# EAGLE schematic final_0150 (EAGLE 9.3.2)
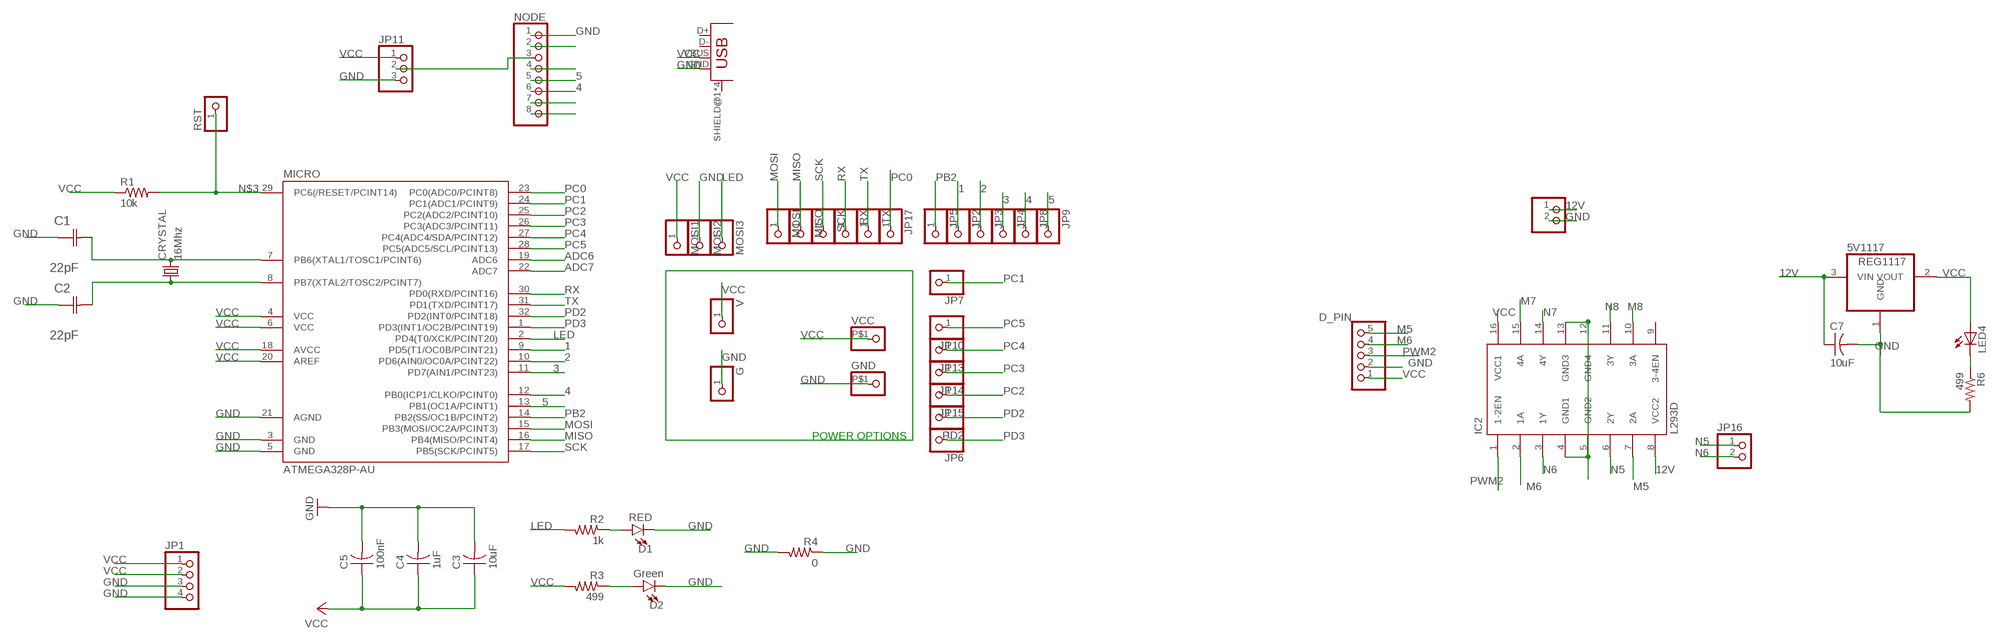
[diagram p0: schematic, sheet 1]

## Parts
5V1117  REG1117  [SOT223]
C1  22pF  0612ZC225MAT2A  [CAPC3216X178N]
C2  22pF  0612ZC225MAT2A  [CAPC3216X178N]
C3  10uF  CAP-US1206FAB  [C1206FAB]
C4  1uF  CAP-US1206FAB  [C1206FAB]
C5  100nF  CAP-US1206FAB  [C1206FAB]
C7  10uF  CAP-US1206FAB  [C1206FAB]
CRYSTAL  16Mhz  CSM-7X-DU  [CSM-7X-DU]
D1  RED  LED-RED1206  [LED-1206]
D2  Green  LED-RED1206  [LED-1206]
D_PIN  PINHD-1X5  [1X05]
G  PINHD-1X1  [1X01]
GND  PINHD-1X1-BIGPOGO  [1X1-BIGPOGO]
IC2  L293D  [DIL16]
JP1  PINHD-1X4  [1X04]
JP2  PINHD-1X1  [1X01]
JP3  PINHD-1X1  [1X01]
JP4  PINHD-1X1  [1X01]
JP5  PINHD-1X1  [1X01]
JP6  PINHD-1X1  [1X01]
JP7  PINHD-1X1  [1X01]
JP8  PINHD-1X1  [1X01]
JP9  PINHD-1X1  [1X01]
JP10  PINHD-1X1  [1X01]
JP11  PINHD-1X3  [1X03]
JP12  PINHD-1X2  [1X02]
JP13  PINHD-1X1  [1X01]
JP14  PINHD-1X1  [1X01]
JP15  PINHD-1X1  [1X01]
JP16  PINHD-1X2  [1X02]
JP17  PINHD-1X1  [1X01]
LED4  LEDSMT1206  [1206]
MICRO  ATMEGA328P-AU  ATMEGA48/88/168-AU  [TQFP32-08]
MISO  PINHD-1X1  [1X01]
MOSI  PINHD-1X1  [1X01]
MOSI1  PINHD-1X1  [1X01]
MOSI2  PINHD-1X1  [1X01]
MOSI3  PINHD-1X1  [1X01]
NODE  PINHD-1X8  [1X08]
PD2  PINHD-1X1  [1X01]
R1  10k  RES-US1206FAB  [R1206FAB]
R2  1k  RES-US1206FAB  [R1206FAB]
R3  499  RES-US1206FAB  [R1206FAB]
R4  0  RES-US1206FAB  [R1206FAB]
R6  499  RESISTOR1206  [1206]
RST  PINHD-1X1  [1X01]
RX  PINHD-1X1  [1X01]
SCK  PINHD-1X1  [1X01]
TX  PINHD-1X1  [1X01]
U$1  USB_MINIB  [USB_MINIB]
V  PINHD-1X1  [1X01]
VCC  PINHD-1X1-BIGPOGO  [1X1-BIGPOGO]

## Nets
1: JP2.1 MICRO.9(PD5(T1/OC0B/PCINT21))
2: JP3.1 MICRO.10(PD6(AIN0/OC0A/PCINT22))
3: JP4.1 MICRO.11(PD7(AIN1/PCINT23))
4: JP8.1 MICRO.12(PB0(ICP1/CLKO/PCINT0)) NODE.6
5: JP9.1 MICRO.13(PB1(OC1A/PCINT1)) NODE.5
12V: 5V1117.3(VIN) C7.1 IC2.8(VCC2) JP12.1
ADC6: MICRO.19(ADC6)
ADC7: MICRO.22(ADC7)
GND: 5V1117.1(GND) C1.1(C1) C2.1(C1) C3.2 C4.2 C5.2 C7.2 D1.C D2.C D_PIN.2 G.1 GND.P$1 IC2.4(GND1) IC2.5(GND2) IC2.12(GND4) IC2.13(GND3) JP1.3 JP1.4 JP11.3 JP12.2 MICRO.3(GND) MICRO.5(GND) MICRO.21(AGND) MOSI2.1 NODE.1 R4.1 R4.2 R6.2 U$1.GND
LED: MICRO.2(PD4(T0/XCK/PCINT20)) MOSI3.1 R2.2
M5: D_PIN.5 IC2.7(2A)
M6: D_PIN.4 IC2.2(1A)
M7: IC2.15(4A)
M8: IC2.10(3A)
MISO: MICRO.16(PB4(MISO/PCINT4)) MISO.1
MOSI: MICRO.15(PB3(MOSI/OC2A/PCINT3)) MOSI.1
N5: IC2.6(2Y) JP16.1
N6: IC2.3(1Y) JP16.2
N7: IC2.14(4Y)
N8: IC2.11(3Y)
N$1: D2.A R3.1
N$2: C1.2(C2) CRYSTAL.2 MICRO.7(PB6(XTAL1/TOSC1/PCINT6))
N$3: MICRO.29(PC6(/RESET/PCINT14)) R1.2 RST.1
N$4: LED4.C R6.1
N$5: NODE.2
N$7: NODE.4
N$8: JP11.2 NODE.3
N$9: C2.2(C2) CRYSTAL.1 MICRO.8(PB7(XTAL2/TOSC2/PCINT7))
N$11: NODE.7
N$12: NODE.8
N$25: D1.A R2.1
PB2: JP5.1 MICRO.14(PB2(SS/OC1B/PCINT2))
PC0: JP17.1 MICRO.23(PC0(ADC0/PCINT8))
PC1: JP7.1 MICRO.24(PC1(ADC1/PCINT9))
PC2: JP15.1 MICRO.25(PC2(ADC2/PCINT10))
PC3: JP14.1 MICRO.26(PC3(ADC3/PCINT11))
PC4: JP13.1 MICRO.27(PC4(ADC4/SDA/PCINT12))
PC5: JP10.1 MICRO.28(PC5(ADC5/SCL/PCINT13))
PD2: MICRO.32(PD2(INT0/PCINT18)) PD2.1
PD3: JP6.1 MICRO.1(PD3(INT1/OC2B/PCINT19))
PWM2: D_PIN.3 IC2.1(1-2EN)
RX: MICRO.30(PD0(RXD/PCINT16)) RX.1
SCK: MICRO.17(PB5(SCK/PCINT5)) SCK.1
TX: MICRO.31(PD1(TXD/PCINT17)) TX.1
VCC: 5V1117.2(VOUT) C3.1 C4.1 C5.1 D_PIN.1 IC2.16(VCC1) JP1.1 JP1.2 JP11.1 LED4.A MICRO.4(VCC) MICRO.6(VCC) MICRO.18(AVCC) MICRO.20(AREF) MOSI1.1 R1.1 R3.2 U$1.VBUS V.1 VCC.P$1
Unconnected: IC2.9(3-4EN) U$1.D+ U$1.D- U$1.SHIELD@1(SHIELD) U$1.SHIELD@2(SHIELD) U$1.SHIELD@3(SHIELD) U$1.SHIELD@4(SHIELD)

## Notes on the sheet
- POWER OPTIONS

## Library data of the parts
5V1117 = burr-brown:REG1117: 800mA and 1A Low Dropout (LDO) Positive Regulator 1.8V, 2.5V, 2.85V, 3.3V, 5V, and Adj; MPN: REG1117; OC_FARNELL: 1097566; OC_NEWARK: 14P6981
C1 C2 = AVX_By_element14_Batch_1:0612ZC225MAT2A: Capacitor 1206; MPN: 0612ZC225MAT2A; OC_FARNELL: -; OC_NEWARK: 12N3209; SUPPLIER: AVX; TOLERANCE: ±20%; VALUE: 2.2µF; VOLTAGERATING: 10V
C3-C5 = fab:CAP-US
C7 = fab (1):CAP-US
CRYSTAL = 01_FAB_Hello:CSM-7X-DU: SMD CRYSTAL; OC_FARNELL: unknown; OC_NEWARK: unknown
D1 = SparkFun-LED:LED-RED: Red SMD LED; PROD_ID: DIO-09912
D2 = SparkFun-LED:LED-RED: Red SMD LED; PROD_ID: DIO-09912; VALUE: RED
D_PIN = pinhead:PINHD-1X5: PIN HEADER
G GND JP2-JP10 JP13-JP15 JP17 MISO MOSI MOSI1-MOSI3 PD2 RST RX SCK TX V VCC = adafruit:PINHD-1X1: Pin header 1x1 for 0.1" spacing
IC2 = st-microelectronics:L293D: PUSH-PULL 4 CHANNEL DRIVER; MPN: L293D; OC_FARNELL: 9589619; OC_NEWARK: 56P8249
JP1 = pinhead:PINHD-1X4: PIN HEADER
JP11 = pinhead:PINHD-1X3: PIN HEADER
JP12 JP16 = pinhead:PINHD-1X2: PIN HEADER
LED4 = led:LED: LED
MICRO = atmega8:ATMEGA48/88/168
NODE = pinhead:PINHD-1X8: PIN HEADER
R1-R4 = fab:RES-US: Resistor (US Symbol)
R6 = 01_SparkFun:RESISTOR: Resistor
U$1 = fab:USB_MINIB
